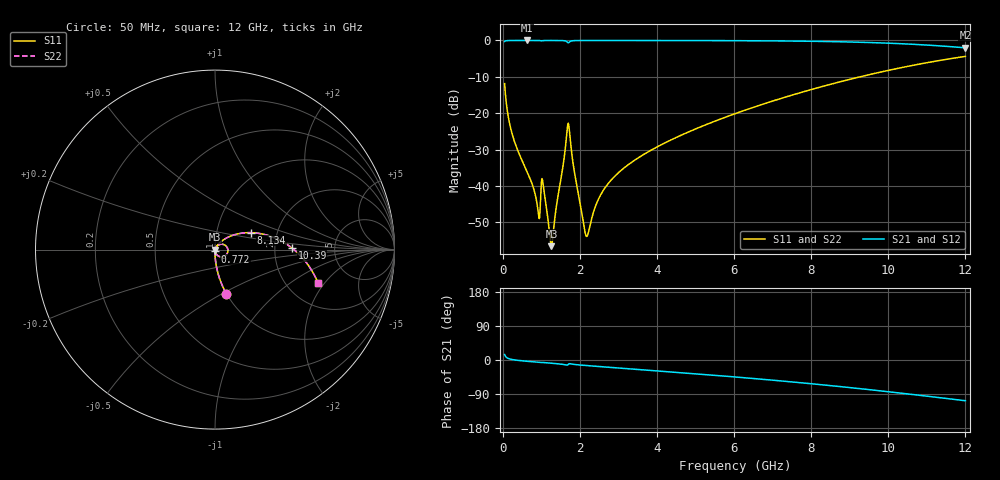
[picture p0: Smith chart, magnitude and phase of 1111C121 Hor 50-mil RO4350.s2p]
# GHz S MA R 50
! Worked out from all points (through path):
!   11951 points, 50 MHz to 12 GHz, reference 50 ohm
!   highest |S21| = -0.01 dB at 625 MHz (marker M1); lowest = -2.0 dB at 12 GHz (marker M2)
!   group delay of S21, straight-line fit = 24.7 ps
!   lowest |S11| = -56.5 dB at 1.263 GHz (marker M3), VSWR 1.00, Z = 50.1 - j0.0225 ohm
!   |S11| at or under -10 dB: start of sweep to 9.268 GHz
!   |S22| runs from -56.5 to -4.4 dB; largest |S21 - S12| = 0
!   S11 on the Smith chart (normalised r, x): 50 MHz: 1.00, -0.53; 772 MHz: 1.00, -0.02; 8.134 GHz: 1.47, +0.29; 10.39 GHz: 2.50, +0.06; 12 GHz: 2.94, -1.73
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0.05  0.2547 -75.5  0.9668 14.4  0.9668 14.4  0.2547 -75.5
0.245  0.05197 -88.2  0.9982 1.3  0.9982 1.3  0.05197 -88.2
0.625  0.01611 -90.9  0.9991 -3.3  0.9991 -3.3  0.01611 -90.9
0.772  0.01033 -90.1  0.9991 -4.6  0.9991 -4.6  0.01033 -90.1
0.923  0.004285 -70.9  0.9981 -6.0  0.9981 -6.0  0.004285 -70.9
1.054  0.01003 -66.8  0.9949 -6.6  0.9949 -6.6  0.01003 -66.8
1.263  0.001491 -8.7  0.9984 -8.5  0.9984 -8.5  0.001491 -8.7
1.694  0.07202 -0.4  0.9293 -12.3  0.9293 -12.3  0.07202 -0.4
1.737  0.05275 -50.8  0.9595 -9.7  0.9595 -9.7  0.05275 -50.8
1.85  0.01683 -79.0  0.9933 -11.6  0.9933 -11.6  0.01683 -79.0
2.042  0.004546 -69.7  0.9973 -13.5  0.9973 -13.5  0.004546 -69.7
2.132  0.002362 -39.2  0.9977 -14.3  0.9977 -14.3  0.002362 -39.2
2.192  0.00206 0.2  0.9979 -14.8  0.9979 -14.8  0.00206 0.2
2.449  0.006006 56.7  0.9981 -16.8  0.9981 -16.8  0.006006 56.7
2.748  0.01101 62.4  0.9981 -19.1  0.9981 -19.1  0.01101 62.4
4.034  0.0351 58.3  0.9974 -28.8  0.9974 -28.8  0.0351 58.3
6.025  0.09847 43.9  0.9925 -44.7  0.9925 -44.7  0.09847 43.9
8.017  0.2126 26.4  0.9736 -62.8  0.9736 -62.8  0.2126 26.4
8.134  0.2212 25.3  0.9716 -63.9  0.9716 -63.9  0.2212 25.3
10.009  0.3886 5.6  0.9167 -83.8  0.9167 -83.8  0.3886 5.6
10.388  0.4281 1.3  0.8988 -88.2  0.8988 -88.2  0.4281 1.3
12  0.6037 -18.0  0.7913 -107.5  0.7913 -107.5  0.6037 -18.0
